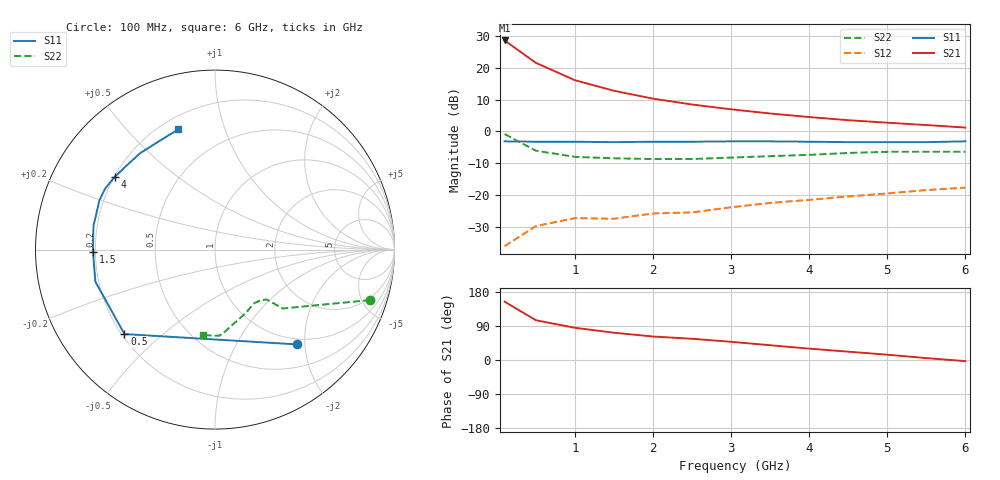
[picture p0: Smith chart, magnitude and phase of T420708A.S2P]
! AT-42070
!S AND NOISE PARAMETERS at Vce=8V  Ic=10mA.  LAST UPDATED 07-21-92
# ghz s ma r 50
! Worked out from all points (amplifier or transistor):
!   13 points, 100 MHz to 6 GHz, reference 50 ohm
!   highest |S21| = 28.5 dB at 100 MHz (marker M1)
!   |S21| within 3 dB of that: start of sweep to 271.2 MHz
!   unconditionally stable (mu >= 1): 1.397 GHz to end of sweep
!   at 1 GHz: K = 0.71, MSG = 21.6 dB, |S12| = -27.1 dB
!   at 3 GHz: K = 1.30, MAG = 12.1 dB, |S12| = -23.7 dB
!   at 6 GHz: K = 1.08, MAG = 7.6 dB, |S12| = -17.6 dB
!   lowest NFmin = 1.00 dB at 100 MHz
!   S11 on the Smith chart (normalised r, x): 100 MHz: 0.89, -1.85; 500 MHz: 0.21, -0.38; 1.5 GHz: 0.19, -0.01; 4 GHz: 0.20, +0.31; 6 GHz: 0.27, +0.70
0.1  0.7 -49.0  26.56 154.0  0.016 77.0  0.91 -18.0
0.5  0.69 -137.0  11.85 105.0  0.033 34.0  0.5 -41.0
1  0.69 -165.0  6.34 85.0  0.044 29.0  0.4 -44.0
1.5  0.68 -179.0  4.33 72.0  0.043 37.0  0.38 -48.0
2  0.69 169.0  3.26 62.0  0.052 42.0  0.37 -54.0
2.5  0.69 164.0  2.64 56.0  0.054 46.0  0.37 -55.0
3  0.7 157.0  2.22 48.0  0.065 52.0  0.39 -63.0
3.5  0.7 151.0  1.91 39.0  0.076 51.0  0.41 -71.0
4  0.69 144.0  1.68 30.0  0.085 55.0  0.43 -77.0
4.5  0.68 137.0  1.5 22.0  0.096 49.0  0.46 -83.0
5  0.68 128.0  1.37 14.0  0.107 50.0  0.48 -87.0
5.5  0.68 117.0  1.26 5.0  0.121 45.0  0.48 -91.0
6  0.7 107.0  1.15 -3.0  0.132 44.0  0.48 -98.0
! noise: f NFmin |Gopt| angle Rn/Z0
0.1  1  0.05  15  0.13
0.5  1.1  0.06  75  0.13
1  1.5  0.1  126  0.12
2  1.9  0.23  172  0.11
4  3  0.45  -145  0.17
